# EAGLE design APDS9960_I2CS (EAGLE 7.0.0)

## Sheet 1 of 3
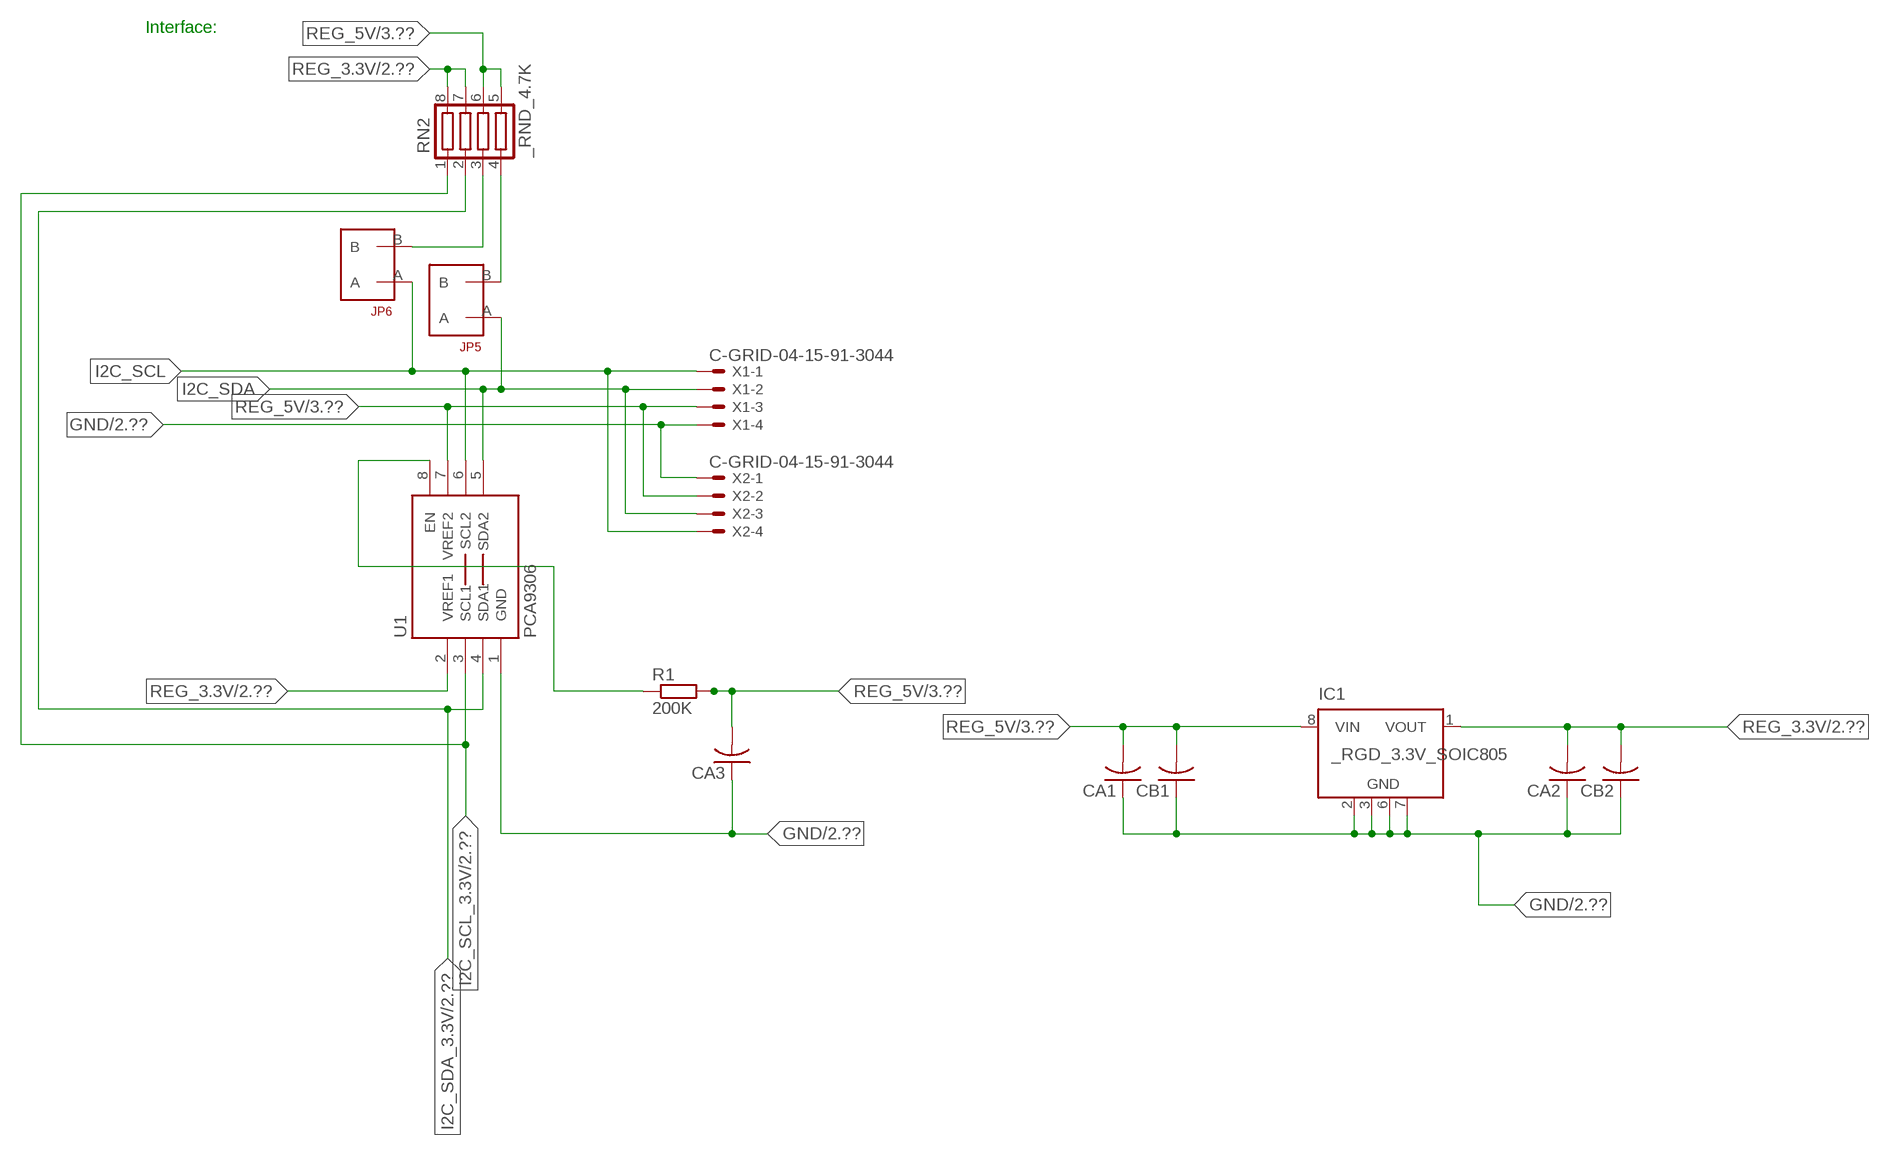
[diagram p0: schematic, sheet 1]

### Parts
CA1  CC1206KRX7R9BB104  [.1UF]
CA2  CC1206KRX7R9BB104  [.1UF]
CA3  CC1206KRX7R9BB104  [.1UF]
CB1  TMK316F106ZL-TC1206K  [TMK316F106ZL-T]
CB2  TMK316F106ZL-TC1206K  [TMK316F106ZL-T]
IC1  _RGD_3.3V_SOIC805  [_RGC_3.3V_SOIC8]
JP5  JUMPER_1X2_2MM  [JUMPER_1X2_2MM]
JP6  JUMPER_1X2_2MM  [JUMPER_1X2_2MM]
R1  200K  RESISTOR_SMT-0603  [R603]
RN2  _RND_4.7K  [RND]
U1  PCA9306  PCA9306_NCD  [PSOP-8]
X1  C-GRID-04-15-91-3044  [15-91-04]
X2  C-GRID-04-15-91-3044  [15-91-04]

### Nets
GND: CA1.1 CA2.1 CA3.1 CB1.1 CB2.1 IC1.2(GND) IC1.3(GND) IC1.6(GND) IC1.7(GND) U1.1(GND) X1.4 X2.1 ; also sheet 2,3
I2C_SCL: JP6.A U1.6(SCL2) X1.1 X2.4
I2C_SCL_3.3V: RN2.1 U1.3(SCL1) ; also sheet 2
I2C_SDA: JP5.A U1.5(SDA2) X1.2 X2.3
I2C_SDA_3.3V: RN2.2 U1.4(SDA1) ; also sheet 2
N$1: JP6.B RN2.3
N$2: JP5.B RN2.4
N$3: R1.1 U1.8(EN)
REG_3.3V: CA2.2 CB2.2 IC1.1(VOUT) RN2.7 RN2.8 U1.2(VREF1) ; also sheet 2
REG_5V: CA1.2 CA3.2 CB1.2 IC1.8(VIN) R1.2 RN2.5 RN2.6 U1.7(VREF2) X1.3 X2.2 ; also sheet 3
Unconnected: IC1.4(NC) IC1.5(NC)

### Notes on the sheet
- Interface:

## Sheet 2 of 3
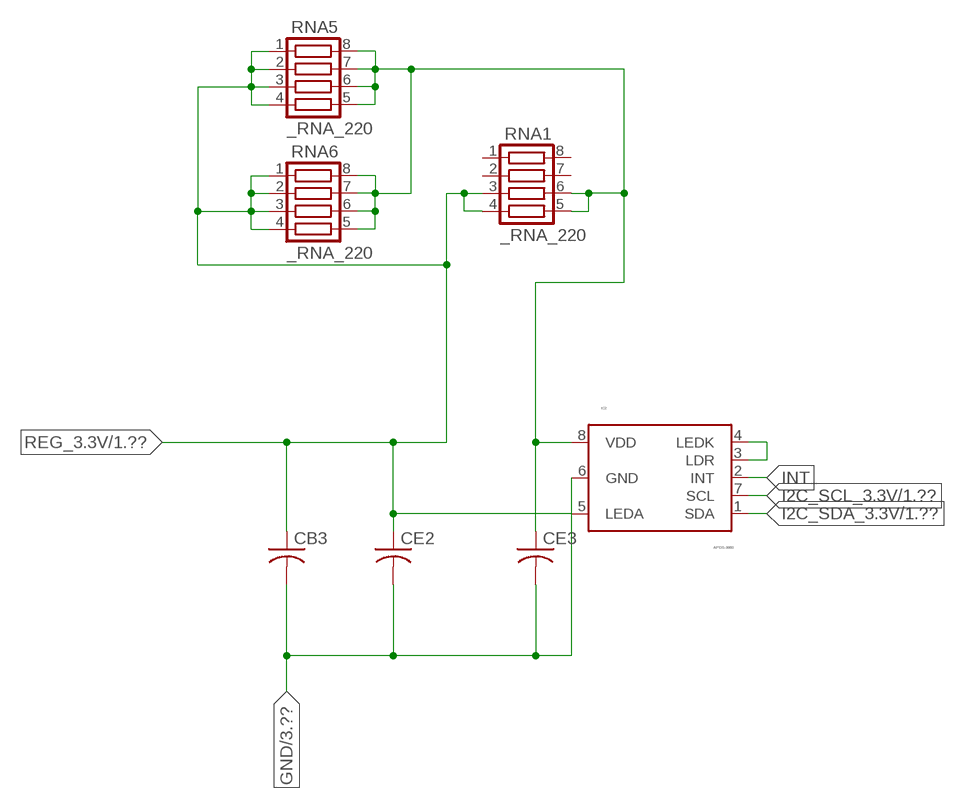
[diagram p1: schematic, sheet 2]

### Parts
CB3  _CB_10UF_25VC1206K  [_CB_10UF_25V]
CE2  CC0603JRNPO8BN1020603  [CC0603JRNPO8BN102]
CE3  CC0603JRNPO8BN1020603  [CC0603JRNPO8BN102]
IC2  APDS-9960  [APDS-9960]
RNA1  _RNA_220  [RNA]
RNA5  _RNA_220  [RNA]
RNA6  _RNA_220  [RNA]

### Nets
GND: CB3.2 CE2.2 CE3.2 IC2.6(GND) ; also sheet 1,3
I2C_SCL_3.3V: IC2.7(SCL) ; also sheet 1
I2C_SDA_3.3V: IC2.1(SDA) ; also sheet 1
INT: IC2.2(INT)
N$7: IC2.3(LDR) IC2.4(LEDK)
REG_3.3V: CB3.1 CE2.1 IC2.5(LEDA) RNA1.3 RNA1.4 RNA5.1 RNA5.2 RNA5.3 RNA5.4 RNA6.1 RNA6.2 RNA6.3 RNA6.4 ; also sheet 1
RNA_22: CE3.1 IC2.8(VDD) RNA1.5 RNA1.6 RNA5.5 RNA5.6 RNA5.7 RNA5.8 RNA6.5 RNA6.6 RNA6.7 RNA6.8
Unconnected: RNA1.1 RNA1.2 RNA1.7 RNA1.8

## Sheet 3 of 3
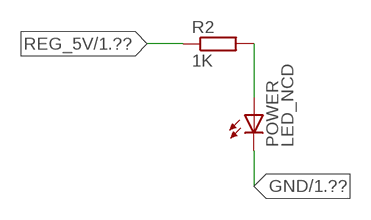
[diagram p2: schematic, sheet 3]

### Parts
POWER  LED_NCD  [CHIPLED_0603]
R2  1K  RESISTOR_SMT-0402  [R402]

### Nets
GND: POWER.C ; also sheet 1,2
N$4: POWER.A R2.2
REG_5V: R2.1 ; also sheet 1

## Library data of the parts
CA1-CA3 = NCD_ULTIMATE_LIBRARY:CC1206KRX7R9BB104: Capacitor CA .1uF 50V SMT C1206K CC1206KRX7R9BB104
CB1 CB2 = NCD_ULTIMATE_LIBRARY:TMK316F106ZL-T: Capacitor CB 10uF SMT 1206 TMK316F106ZL-T
CB3 = NCD_ULTIMATE_LIBRARY (1):_CB_10UF_25V: Capacitor 10uF SMT
CE2 CE3 = NCD_ULTIMATE_LIBRARY (1):CC0603JRNPO8BN102: Capacitor CE 1uF SMT CC0603JRNPO8BN102 0603
IC1 = NCD_ULTIMATE_LIBRARY:_RGD_3.3V_SOIC8: Regulator Linear 3.3V Chip Positive VOLTAGE REGULATOR Digikey 497-1199-2-ND/L78L33ACD13TR
IC2 = NCD_ULTIMATE_KAMNA:APDS-9960: Avago APDS-9960 digital proximity, ambient light, RGB, and gesture sensor.; PROD_ID: SEN-12005
JP5 JP6 = NCD_ULTIMATE_CONNECTORS:JUMPER_1X2_2MM
POWER = NCD_ULTIMATE_LIBRARY:LED_NCD: LED Digikey 754-1132-2-ND/APT2012SRCPRV
R1 R2 = NCD_ULTIMATE_LIBRARY:RESISTOR_SMT: NCD Resistor
RN2 = NCD_ULTIMATE_LIBRARY:_RND_4.7K: Resistor Array RND SMT 4.7K x 4 Single Resistor Source: http://www.ctscorp.com/components/Datasheets/CTSChipArrayDs.pdf Digikey 742C083472JPTR-ND/742C083472JP; OC_FARNELL: unknown; OC_NEWARK: unknown
RNA1 RNA5 RNA6 = NCD_ULTIMATE_LIBRARY (1):_RNA_220: Resistor Array RNA SMT 220 x 4 Single Resistor Source: http://www.ctscorp.com/components/Datasheets/CTSChipArrayDs.pdf Digikey 742C083221JPTR-ND/742C083221JP; OC_FARNELL: unknown; OC_NEWARK: unknown
U1 = NCD_ULTIMATE_LIBRARY:PCA9306_NCD: NCD Bidirectional I2C level shifter. NOT compatible with all available part number pinout schemes- DOUBLE CHECK!!!; PROD_ID: IC-10023
X1 X2 = NCD_ULTIMATE_CONNECTORS:C-GRID-04: CONNECTOR 4-Pos I2C wire to board 2.54 mm (0.100") pitch header Digikey WM1342-ND/0015912045; OC_FARNELL: unknown; OC_NEWARK: unknown

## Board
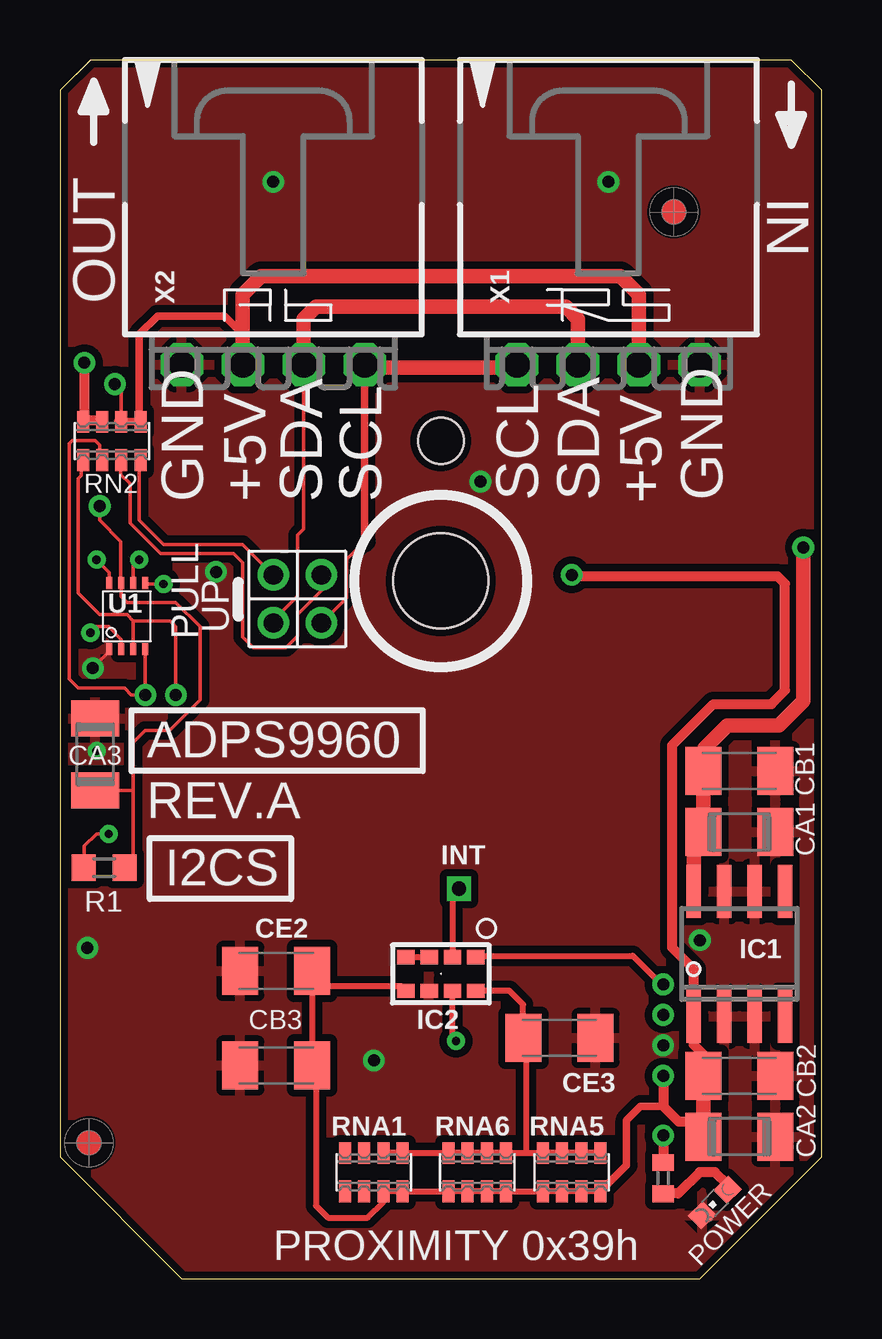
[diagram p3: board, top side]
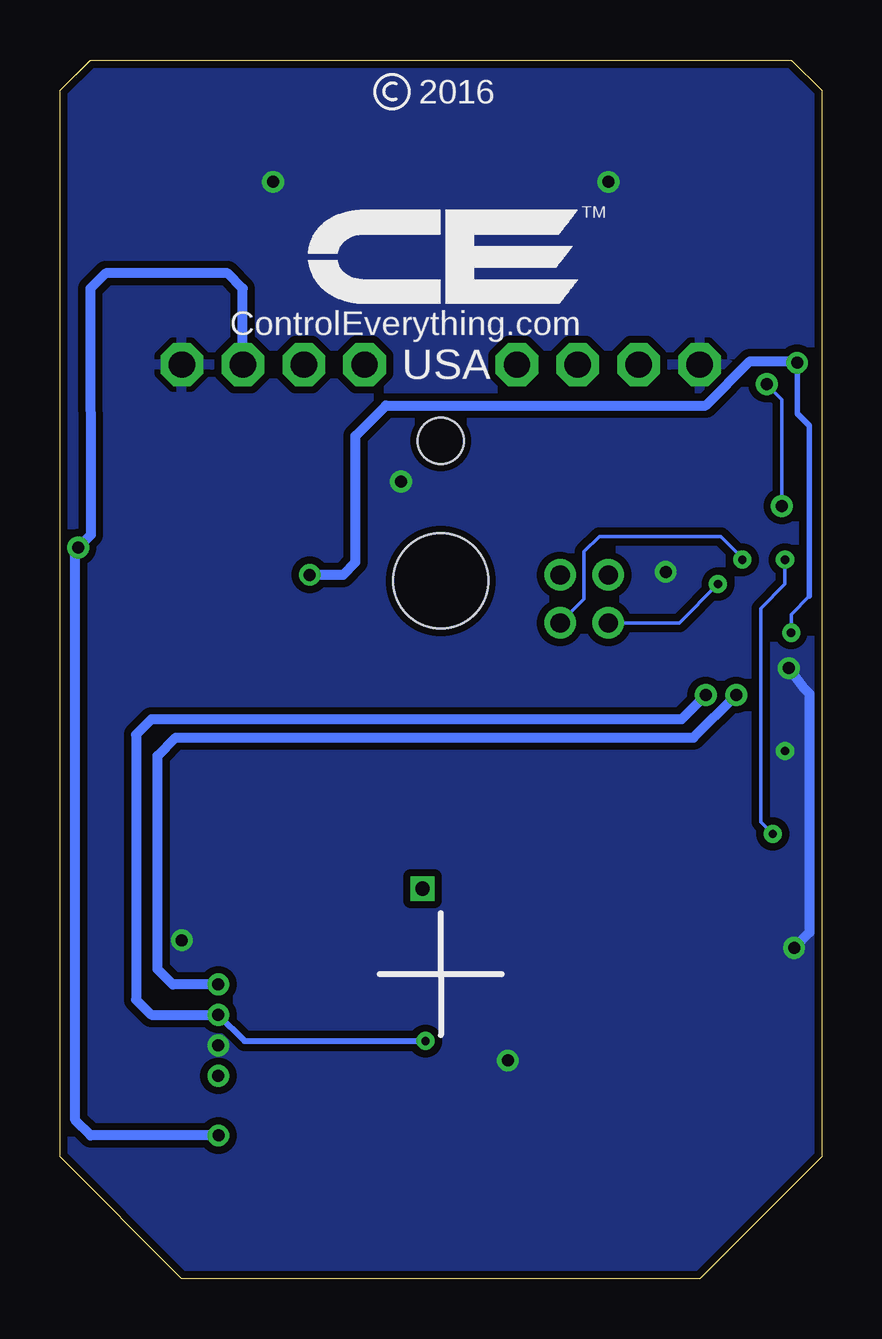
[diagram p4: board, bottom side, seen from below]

Size 31.75 x 50.8 mm. Coordinates in mm from the lower left corner, seen from the top.
Outline: 32 segments
Copper layers (1*16): Top 0.035mm / dielectric 1.5mm / Bottom 0.035mm
Design rules "default": minimum track width 5mil, minimum drill 24mil, track to track 5mil, track to pad 5mil, pad to pad 5mil, via to via 5mil, smd to smd 5mil, copper to edge 10mil, drill to drill 8mil, minimum pad ring 10mil, minimum via ring 8mil, stop-mask expansion 2mil, vias tented up to drill 0mil, thermal gap 10mil
Holes 3.96 mm at 15.88,29.08
Holes 1.91 mm at 15.88,34.93

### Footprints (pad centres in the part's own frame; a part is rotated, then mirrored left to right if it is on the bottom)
.1UF = smd 1.5 x 2: 1 -1.5,0; 2 1.5,0
TMK316F106ZL-T = smd 1.5 x 2: 1 -1.5,0; 2 1.5,0
_CB_10UF_25V = smd 1.5 x 2: 1 -1.5,0; 2 1.5,0
CC0603JRNPO8BN102 = smd 1.5 x 2: 1 -1.5,0; 2 1.5,0
_RGC_3.3V_SOIC8 = smd 0.6 x 2.2: 1 -1.905,-2.6; 2 -0.635,-2.6; 3 0.635,-2.6; 4 1.905,-2.6; 5 1.905,2.6; 6 0.635,2.6; 7 -0.635,2.6; 8 -1.905,2.6
APDS-9960 = smd 0.6 x 0.72: 1 -0.7,1.455; 2 -0.7,0.485; 3 -0.7,-0.485; 4 -0.7,-1.455; 5 0.7,-1.455; 6 0.7,-0.485; 7 0.7,0.485; 8 0.7,1.455
JUMPER_1X2_2MM = drill 0.8: A 0,2; B 0,0
CHIPLED_0603 = smd 0.8 x 0.876: A 0,-0.75; C 0,0.75
R603 = smd 1 x 1.1: 1 -0.85,0; 2 0.85,0
R402 = smd 0.7 x 0.9: 1 -0.65,0; 2 0.65,0
RND = smd 0.5 x 0.9: 1 -1.2,-0.8; 2 -0.4,-0.8; 3 0.4,-0.8; 4 1.2,-0.8; 5 1.2,0.8; 6 0.4,0.8; 7 -0.4,0.8; 8 -1.2,0.8
RNA = smd 0.5 x 0.9: 1 -1.2,-0.8; 2 -0.4,-0.8; 3 0.4,-0.8; 4 1.2,-0.8; 5 1.2,0.8; 6 0.4,0.8; 7 -0.4,0.8; 8 -1.2,0.8
PSOP-8 = smd 0.25 x 0.5: 1 -0.73,-1.37; 2 -0.23,-1.37; 3 0.27,-1.37; 4 0.77,-1.37; 5 0.77,1.38; 6 0.27,1.38; 7 -0.23,1.38; 8 -0.73,1.38
15-91-04 = drill 1.1 pad 1.778 octagon: 1 -3.81,-7.62; 2 -1.27,-7.62; 3 1.27,-7.62; 4 3.81,-7.62

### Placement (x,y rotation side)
CA1  28.32,18.62 180 top
CA2  28.32,5.92 180 top
CA3  1.46,21.86 270 top
CB1  28.32,21.16 180 top
CB2  28.32,8.46 180 top
CB3  9.02,8.89 180 top
CE2  9.02,12.83 180 top
CE3  20.83,10.03 0 top
IC1  28.32,13.54 0 top
IC2  15.88,12.7 270 top
JP5  8.89,29.34 180 top
JP6  10.9,29.34 180 top
POWER  27.3,3.18 135 top
R1  1.84,17.13 0 top
R2  25.15,4.19 270 top
RN2  2.16,34.93 0 top
RNA1  13.08,4.45 0 top
RNA5  21.34,4.45 0 top
RNA6  17.4,4.45 0 top
U1  2.79,27.61 0 top
U$5  [VISION_REF10]  1.21,5.66 90 top
U$28  [VISION_REF10]  25.59,44.46 90 top
X1  22.86,45.72 0 top
X2  8.89,45.72 0 top

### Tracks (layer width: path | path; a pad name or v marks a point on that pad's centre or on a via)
GND  (via drill 0.35, 0.5)
  Top 0.152: CA3.1 1.52,23.42 1.52,23.62 | v1.37,25.45 2.06,26.14 U1.1
  Bottom 0.406: v1.37,25.45 0.76,24.64 0.51,24.38 0.51,14.43 v1.15,13.79
  other vias: 8.89,45.72 22.86,45.72 25.15,9.73 17.53,33.22 26.67,14.11 6.5,29.46 13.08,9.09 1.52,22
  pour Bottom (isolate 0.305): -0.64,5.08 -0.64,49.53 1.27,51.44 30.48,51.44 32.38,49.53 32.38,5.08 26.67,-0.63 5.08,-0.63
  pour Top (isolate 0.305): 4.45,-1.27 -1.27,4.45 -1.27,50.17 0.64,52.07 31.11,52.07 33.02,50.17 33.02,4.45 27.3,-1.27
I2C_SCL  (via drill 0.35)
  Top 0.152: 12.7,30.73 11.94,29.97 11.94,28.38 JP6.A | v3.3,29.97 3.06,29.73 U1.6
  Top 0.305: 12.7,30.73 X2.4
  Top 0.406: X2.4 12.7,37.97 | 19.05,37.97 X1.1
  Top 0.61: 12.7,37.97 19.05,37.97
  Bottom 0.152: JP6.A 9.91,28.33 9.91,30.3 9.27,30.94 4.19,30.94 3.3,30.05 v3.3,29.97
I2C_SCL_3.3V  (via drill 0.35, 0.5)
  Top 0.152: RN2.1 0.89,34.07 0.89,33.48 0.77,33.35 0.77,28.59 1.67,27.69 2.79,27.69 3.06,27.42 | 3.06,27.42 U1.3 | v4.83,24.33 v4.83,24.34 4.83,27.18 4.58,27.42 3.06,27.42
  Top 0.254: v16.51,9.91 16.36,10.06 IC2.7
  Bottom 0.254: v25.15,11 24.06,9.91 v16.51,9.91
  Bottom 0.406: v4.83,24.33 5.84,23.32 27.94,23.32 28.58,22.68 28.58,11.63 27.94,11 v25.15,11
I2C_SDA  (via drill 0.35)
  Top 0.152: JP5.A 8.89,27.44 9.91,28.45 9.91,30.99 10.16,31.24 10.16,34.92 X2.3 | U1.5 3.6,28.96 v4.32,28.96
  Top 0.61: X2.3 10.16,40.01 10.67,40.51 21.09,40.51 21.59,40.01 X1.2
  Bottom 0.152: v4.32,28.96 5.94,27.34 JP5.A
I2C_SDA_3.3V  (via drill 0.5)
  Top 0.152: RN2.2 1.65,34.14 1.65,34.75 1.46,34.94 0.51,34.94 0.38,34.81 0.38,26.37 0.38,26.36 0.38,24.99 0.76,24.61 2.69,24.61 2.97,24.33 v3.56,24.33 U1.4
  Top 0.254: IC2.1 17.39,13.46 23.88,13.46 25.07,12.27 v25.15,12.27
  Bottom 0.406: v25.15,12.27 27.05,12.27 27.69,12.9 27.69,21.79 26.93,22.56 5.34,22.56 v3.56,24.33
INT  (via drill 0.6)
  Top 0.254: v16.64,16.26 16.36,15.98 IC2.2
N$1
  Top 0.152: JP6.B 10.92,29.31 10.92,28.7 9.91,27.69 9.91,26.8 9.42,26.31 8.06,26.31 7.62,26.75 7.62,29.84 7.24,30.23 4.19,30.23 2.92,31.5 2.92,33.15 2.54,33.53 2.54,34.1 RN2.3
  Top 0.305: 2.54,34.02 RN2.3
N$2
  Top 0.152: JP5.B 7.62,30.61 4.32,30.61 3.3,31.62 3.3,34.07 RN2.4
  Top 0.305: 3.37,33.88 RN2.4
N$3  (via drill 0.35)
  Top 0.152: R1.1 1.02,17.16 1.02,18.03 1.52,18.54 v2.03,18.54 | v1.52,29.97 2.06,29.44 U1.8
  Bottom 0.152: v2.03,18.54 2.54,19.05 2.54,27.94 1.52,28.96 v1.52,29.97
N$4
  Top 0.406: POWER.A 27.84,3.92 27.3,4.45 26.67,4.45 25.78,3.56 25.16,3.56 R2.2
N$7
  Top 0.254: IC2.3 IC2.4
REG_3.3V  (via drill 0.35, 0.5)
  Top 0.152: v1.27,26.92 1.52,27.18 2.03,27.18 2.56,26.65 U1.2
  Top 0.254: 10.52,12.19 CE2.1 10.52,12.93 10.92,13.34 | 10.52,12.19 CB3.1 10.67,8.74 10.67,3.05 11.18,2.54 12.83,2.54 13.48,3.19 RNA1.3 RNA1.4 RNA6.1 RNA6.2 RNA6.3 RNA6.4 RNA5.1 RNA5.2 RNA5.3 RNA5.4 | 26.82,5.49 CA2.2 | IC2.5 14.23,12.19 10.52,12.19
  Top 0.305: RNA5.4 23.62,4.73 23.62,6.6 24.21,7.19 25.15,7.19
  Top 0.406: CB2.2 26.82,9.35 26.42,9.75 26.42,10.36 | v25.15,8.46 25.15,7.19 25.78,6.55 26.82,6.55 | IC1.1 26.42,12.9 25.53,13.79 25.53,22.24 27.24,23.95 29.66,23.95 30.23,24.52 30.23,28.97 29.91,29.29 21.39,29.29 v21.34,29.34 | 26.52,5.62 CA2.2 | v1.02,38.18 1.02,35.78 | 1.02,35.78 RN2.8 | 1.02,35.78 1.71,35.78 RN2.7
  Top 0.61: CB2.2 26.82,6.55 CA2.2 | 26.42,10.36 IC1.1
  Bottom 0.152: 0.51,28.45 1.27,27.69 v1.27,26.92
  Bottom 0.229: 0.51,28.45 0.51,35.56 1.02,36.07 v1.02,38.18
  Bottom 0.406: v1.02,38.18 1.08,38.24 2.99,38.24 4.83,36.4 18.16,36.4 19.43,35.13 19.43,29.87 19.94,29.34 v21.34,29.34
REG_5V  (via drill 0.5)
  Top 0.152: RN2.6 2.56,37.01 v2.29,37.29 | R1.2 3.05,17.49 3.05,20.36 | 3.05,20.36 3.05,22.35 3.56,22.86 4.57,22.86 5.84,24.13 5.84,27.18 4.83,28.19 2.79,28.19 2.56,28.43 U1.7 2.54,29.01 2.54,30.73 1.65,31.62 v1.65,32.21 | CA3.2 3.05,20.36
  Top 0.305: 7.62,39.37 7.5,39.37 | 2.42,35.74 RN2.6 RN2.5 3.31,35.8 3.31,39.37 4.07,40.13 6.86,40.13 7.62,39.37 | X2.2 7.62,39.37
  Top 0.406: v25.15,5.97 R2.1
  Top 0.61: X1.3 24.13,41.02 23.37,41.78 8.38,41.78 7.62,41.02 X2.2 | IC1.8 26.42,18.21 CA1.2 CB1.2 26.86,21.2 26.86,22.11 27.82,23.06 29.98,23.06 30.99,24.08 v30.99,30.48
  Bottom 0.152: v1.65,32.21 1.65,36.65 v2.29,37.29
  Bottom 0.406: X1.3 24.13,41.28 24.77,41.91 29.84,41.91 30.48,41.27 30.47,31 v30.99,30.48 31.11,30.36 31.11,6.6 30.48,5.97 v25.15,5.97
RNA_22
  Top 0.254: RNA5.5 RNA5.6 RNA5.7 RNA5.8 19.43,5.25 | RNA1.6 RNA1.5 RNA6.8 RNA6.7 RNA6.6 RNA6.5 19.43,5.25 | 19.43,5.25 19.43,9.93 CE3.1 19.3,10.06 19.3,11.43 18.73,12 IC2.8

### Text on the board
tNames: IN | OUT | GND | +5V | SDA | SCL | SCL | SDA | +5V | GND | PULL | UP | ADPS9960 | REV.A | INT | I2CS | PROXIMITY 0x39h
bNames: 2016 | TM | ControlEverything.com | USA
